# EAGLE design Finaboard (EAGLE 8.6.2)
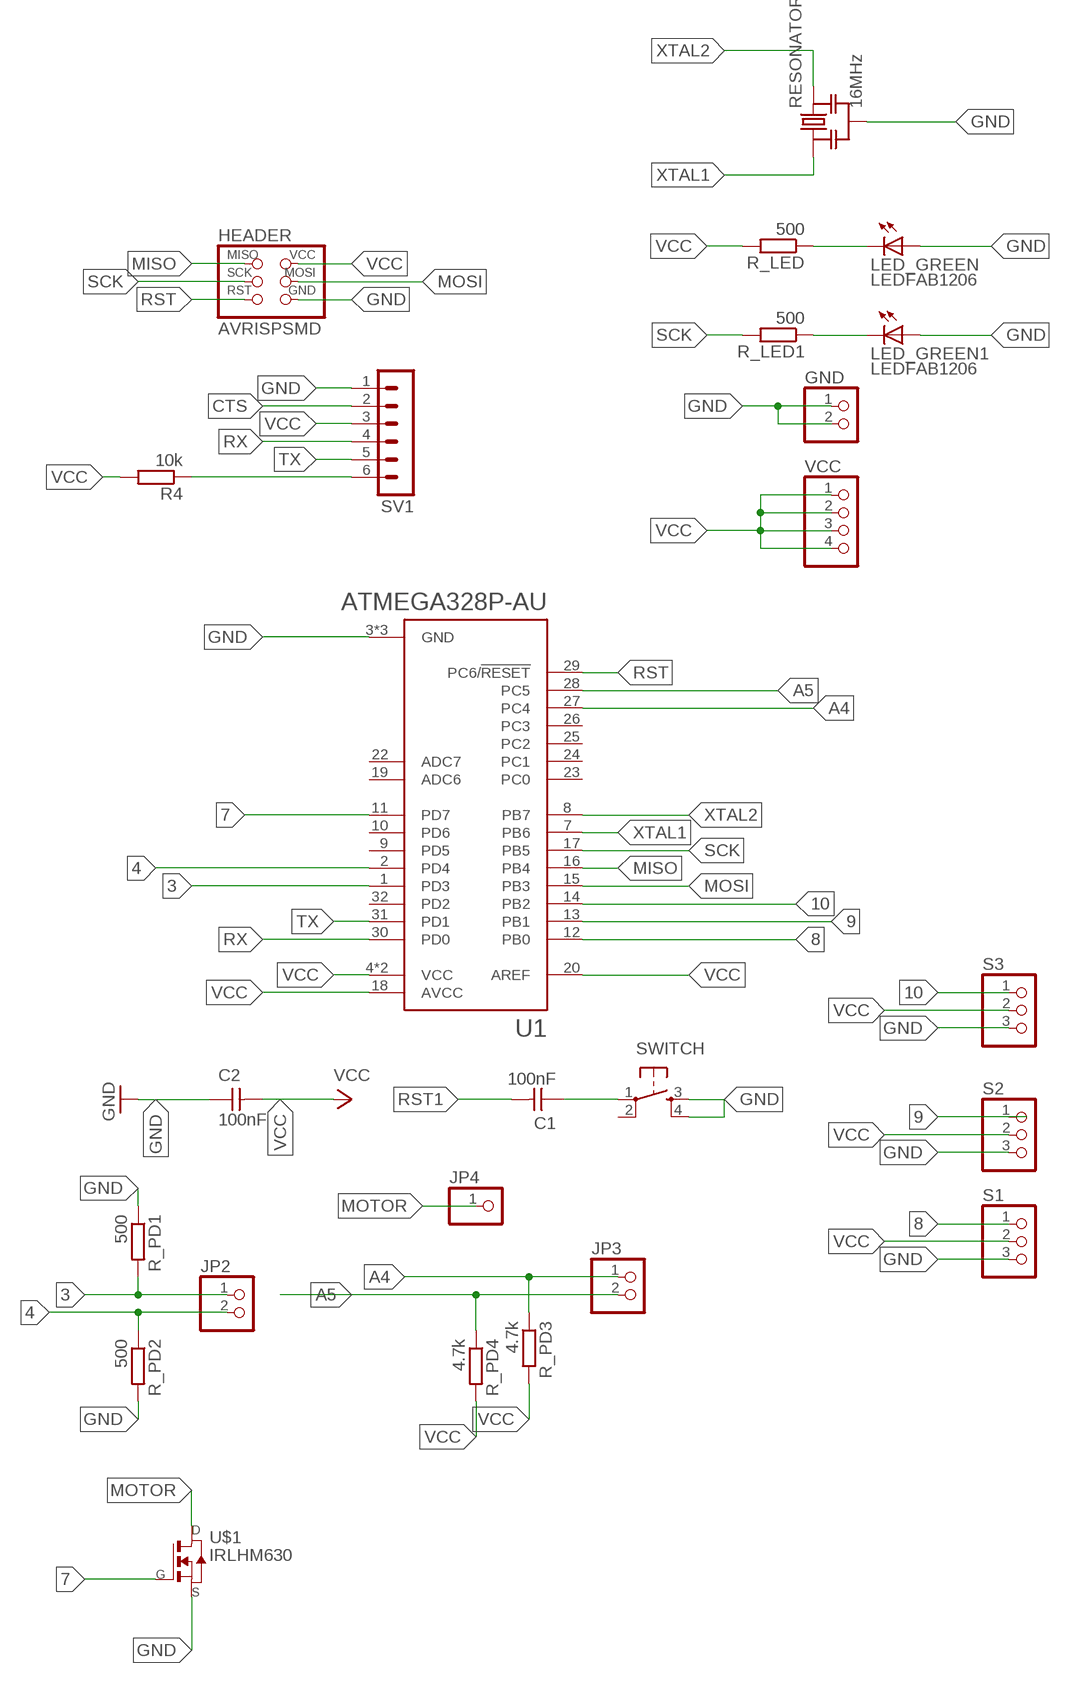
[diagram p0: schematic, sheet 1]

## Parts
C1  100nF  CAP-UNPOLARIZEDFAB  [C1206FAB]
C2  100nF  CAP-UNPOLARIZEDFAB  [C1206FAB]
GND  PINHD-1X2  [1X02]
HEADER  AVRISPSMD  [2X03SMD]
JP2  PINHD-1X2  [1X02]
JP3  PINHD-1X2  [1X02]
JP4  PINHD-1X1  [1X01]
LED_GREEN  LEDFAB1206  [LED1206FAB]
LED_GREEN1  LEDFAB1206  [LED1206FAB]
R4  10k  R-EU_R1206  [R1206]
R_LED  500  R-EU_R1206  [R1206]
R_LED1  500  R-EU_R1206  [R1206]
R_PD1  500  R-EU_R1206  [R1206]
R_PD2  500  R-EU_R1206  [R1206]
R_PD3  4.7k  R-EU_R1206  [R1206]
R_PD4  4.7k  R-EU_R1206  [R1206]
RESONATOR  16MHz  RESONATOR-MURATACSTCR_G  [RESONATOR_MURATA3]
S1  PINHD-1X3  [1X03]
S2  PINHD-1X3  [1X03]
S3  PINHD-1X3  [1X03]
SV1  MA06-1  [MA06-1]
SWITCH  6MM_SWITCH6MM_SWITCH  [6MM_SWITCH]
U1  ATMEGA328P-AU  [QFP80P900X900X120-32N]
U$1  IRLHM630  [IRF-PQFN3.3X3.3B]
VCC  PINHD-1X4  [1X04]

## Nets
3: JP2.1 R_PD1.2 U1.1(PD3)
4: JP2.2 R_PD2.1 U1.2(PD4)
7: U1.11(PD7) U$1.G
8: S1.1 U1.12(PB0)
9: S2.1 U1.13(PB1)
10: S3.1 U1.14(PB2)
A4: JP3.1 R_PD3.1 U1.27(PC4)
A5: JP3.2 R_PD4.1 U1.28(PC5)
CTS: SV1.2
GND: C2.1 GND.1 GND.2 HEADER.6(GND) LED_GREEN1.1(A) LED_GREEN.1(A) R_PD1.1 R_PD2.2 RESONATOR.2 S1.3 S2.3 S3.3 SV1.1 SWITCH.3(S) SWITCH.4(S1) U1.3(GND) U1.5(GND) U1.21(GND) U$1.S
MISO: HEADER.1(MISO) U1.16(PB4)
MOSI: HEADER.4(MOSI) U1.15(PB3)
MOTOR: JP4.1 U$1.D
N$1: LED_GREEN1.2(C) R_LED1.1
N$21: LED_GREEN.2(C) R_LED.1
RST: C1.1 HEADER.5(RST) SWITCH.1(P) U1.29(PC6/!RESET)
RST1: C1.2 R4.1 SV1.6
RX: SV1.4 U1.30(PD0)
SCK: HEADER.3(SCK) R_LED1.2 U1.17(PB5)
TX: SV1.5 U1.31(PD1)
VCC: C2.2 HEADER.2(VCC) R4.2 R_LED.2 R_PD3.2 R_PD4.2 S1.2 S2.2 S3.2 SV1.3 U1.4(VCC) U1.6(VCC) U1.18(AVCC) U1.20(AREF) VCC.1 VCC.2 VCC.3 VCC.4
XTAL1: RESONATOR.1 U1.7(PB6)
XTAL2: RESONATOR.3 U1.8(PB7)
Unconnected: SWITCH.2(P1) U1.9(PD5) U1.10(PD6) U1.19(ADC6) U1.22(ADC7) U1.23(PC0) U1.24(PC1) U1.25(PC2) U1.26(PC3) U1.32(PD2)

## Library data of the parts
C1 C2 = fab:CAP-UNPOLARIZED
GND JP2 JP3 = pinhead:PINHD-1X2: PIN HEADER
HEADER = fab:AVRISP
JP4 = pinhead:PINHD-1X1: PIN HEADER
LED_GREEN LED_GREEN1 = fab:LED: LED
R4 R_LED R_LED1 R_PD1-R_PD4 = resistor:R-EU_: RESISTOR, European symbol
RESONATOR = m-pad-2.1:RESONATOR-MURATA: Murata ceramic Resonator "ceralock" CSTCE series with built in load capacitance +- 0.5% tolerance 12.51MHz to 19.99MHz 16MHz murata part#: CSTCE16M0V53-R0 16MHz digikey part#: 490-1198-1-ND $1.33 each
S1-S3 = pinhead:PINHD-1X3: PIN HEADER
SV1 = con-lstb:MA06-1: PIN HEADER; OC_FARNELL: unknown; OC_NEWARK: unknown
SWITCH = fab:6MM_SWITCH: OMRON SWITCH
U1 = ATMEGA328P-AU:ATMEGA328P-AU: ATmega Series 20 MHz 32 KB Flash 2 KB SRAM 8-Bit Microcontroller - TQFP-32; AVAILABILITY: Good; DESCRIPTION: ATmega Series 20 MHz 32 KB Flash 2 KB SRAM 8-Bit Microcontroller - TQFP-32; MF: Atmel; MP: ATMEGA328P-AU; PACKAGE: TQFP-32 Atmel; PRICE: 2.38 USD
U$1 = fab:IRLHM630
VCC = pinhead:PINHD-1X4: PIN HEADER

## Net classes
0 default: clearance 0.205 mm

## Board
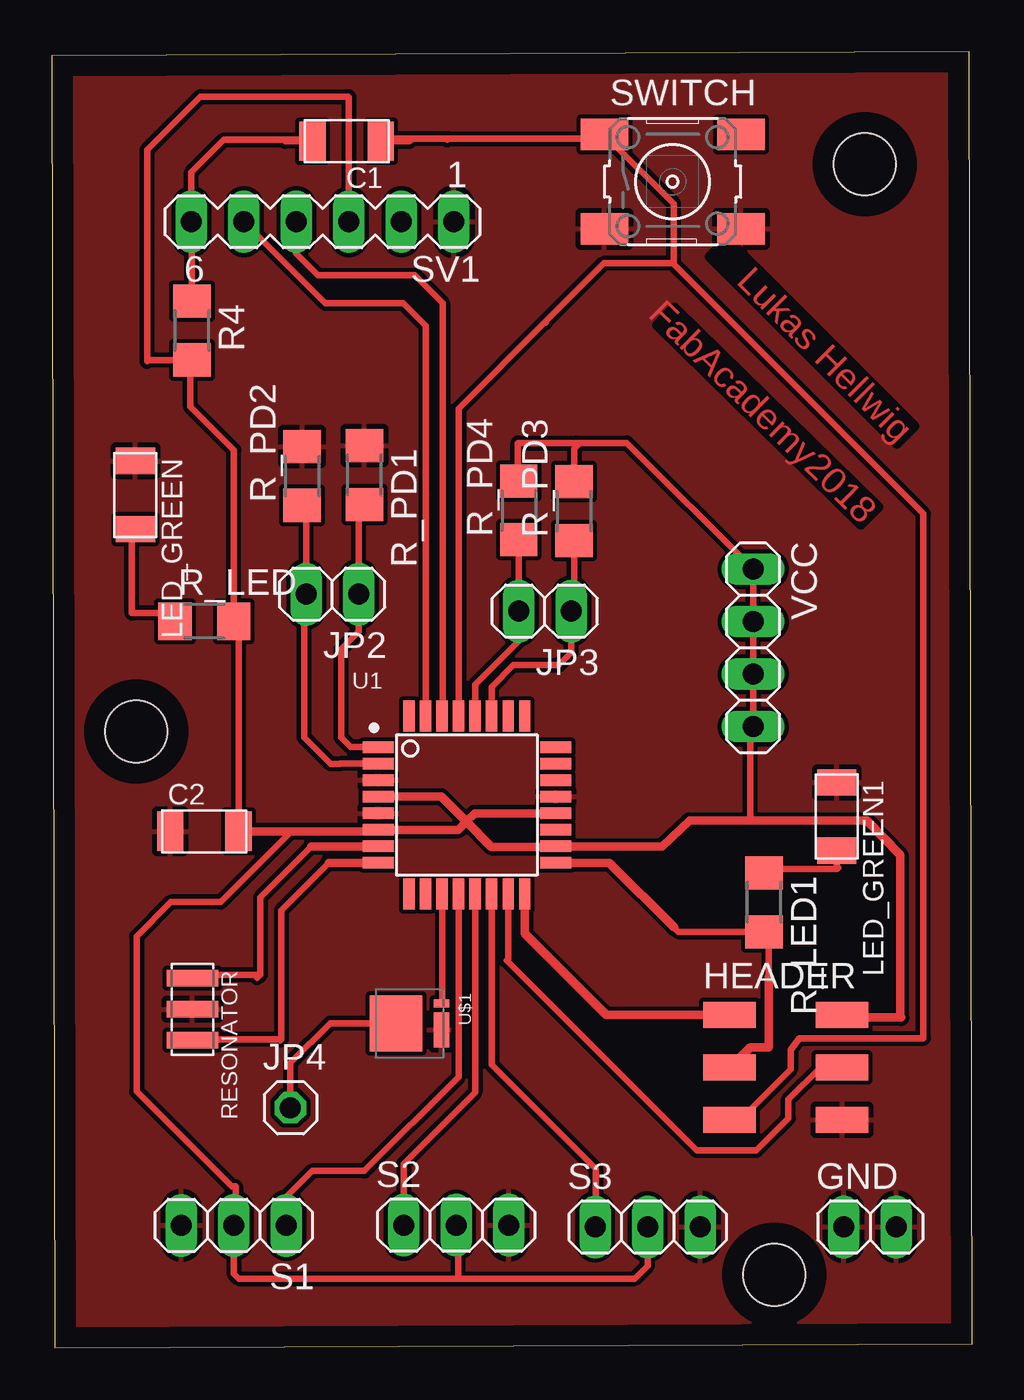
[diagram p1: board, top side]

Size 44.53 x 62.74 mm. Coordinates in mm from the lower left corner, seen from the top.
Outline: 0.14,0 44.53,0.2 44.39,62.74 0,62.54 0.14,0
Copper layers (1*16): Top 0.035mm / dielectric 1.5mm / Bottom 0.035mm
Design rules "default *": minimum track width 6mil, minimum drill 0.35mm, track to track 8mil, track to pad 8mil, pad to pad 8mil, via to via 8mil, smd to smd 8mil, copper to edge 40mil, drill to drill 8mil, minimum pad ring 10mil, minimum via ring 8mil, stop-mask expansion 4mil, vias tented up to drill 0mil, thermal gap 10mil
Holes 3 mm at 39.34,57.3 34.96,3.54 4.09,29.84

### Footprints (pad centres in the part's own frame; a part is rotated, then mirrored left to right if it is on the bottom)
C1206FAB = smd 1.27 x 1.905: 1 -1.651,0; 2 1.651,0
1X02 = drill 1.016 long: 1 -1.27,0; 2 1.27,0
2X03SMD = smd 2.54 x 1.27: 1 -2.54,2.54; 2 2.92,2.54; 3 -2.54,0; 4 2.92,0; 5 -2.54,-2.54; 6 2.92,-2.54
1X01 = drill 1.016 octagon: 1 0,0
LED1206FAB = smd 1.27 x 1.905: 1 -1.651,0; 2 1.651,0
R1206 = smd 1.6 x 1.803: 1 -1.422,0; 2 1.422,0
RESONATOR_MURATA3 = smd 0.8 x 2.5: 1 -1.5,0; 2 0,0; 3 1.5,0
1X03 = drill 1.016 long: 1 -2.54,0; 2 0,0; 3 2.54,0
MA06-1 = drill 1.016 long: 1 -6.35,0; 2 -3.81,0; 3 -1.27,0; 4 1.27,0; 5 3.81,0; 6 6.35,0
6MM_SWITCH = smd 2.286 x 1.524: 1 -3.302,2.286; 2 3.302,2.286; 3 -3.302,-2.286; 4 3.302,-2.286
QFP80P900X900X120-32N = smd 1.5 x 0.55: 1 -4.3,2.8; 2 -4.3,2; 3 -4.3,1.2; 4 -4.3,0.4; 5 -4.3,-0.4; 6 -4.3,-1.2; 7 -4.3,-2; 8 -4.3,-2.8; 17 4.3,-2.8; 18 4.3,-2; 19 4.3,-1.2; 20 4.3,-0.4; 21 4.3,0.4; 22 4.3,1.2; 23 4.3,2; 24 4.3,2.8 | smd 0.55 x 1.5: 9 -2.8,-4.3; 10 -2,-4.3; 11 -1.2,-4.3; 12 -0.4,-4.3; 13 0.4,-4.3; 14 1.2,-4.3; 15 2,-4.3; 16 2.8,-4.3; 25 2.8,4.3; 26 2,4.3; 27 1.2,4.3; 28 0.4,4.3; 29 -0.4,4.3; 30 -1.2,4.3; 31 -2,4.3; 32 -2.8,4.3
IRF-PQFN3.3X3.3B = smd 2.7 x 2.54: D 0,-1.27 | smd 0.39 x 0.77: G -0.975,0.925 | smd 1.69 x 0.77: S 0.325,0.925
1X04 = drill 1.016 long: 1 -3.81,0; 2 -1.27,0; 3 1.27,0; 4 3.81,0

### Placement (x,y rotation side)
C1  14.27,58.41 180 top
C2  7.39,25.01 0 top
GND  39.6,5.85 0 top
HEADER  35.33,13.58 0 top
JP2  13.58,36.48 180 top
JP3  23.87,35.65 180 top
JP4  11.55,11.63 0 top
LED_GREEN  4.05,41.28 270 top
LED_GREEN1  37.99,25.72 270 top
R4  6.79,49.25 270 top
R_LED  7.39,35.17 0 top
R_LED1  34.47,21.56 270 top
R_PD1  15.13,42.25 270 top
R_PD2  12.12,42.21 90 top
R_PD3  25.28,40.5 90 top
R_PD4  22.6,40.54 90 top
RESONATOR  6.81,16.39 270 top
S1  8.81,5.93 180 top
S2  19.57,5.94 0 top
S3  28.84,5.85 0 top
SV1  13.11,54.51 180 top
SWITCH  30.05,56.45 0 top
U1  20.09,26.28 0 top
U$1  17.94,15.71 270 top
VCC  33.94,33.88 270 top

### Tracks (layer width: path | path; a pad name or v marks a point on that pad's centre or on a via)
3
  Top 0.305: U1.1 14.48,29.08 14,29.55 14,33.83 14.85,34.68 JP2.1 14.85,40.55 R_PD1.2
4
  Top 0.305: U1.2 13.96,28.28 13.95,28.27 13.49,28.27 12.21,29.55 12.21,36.38 JP2.2 12.31,40.59 R_PD2.1
7
  Top 0.305: U1.11 18.89,16.71 U$1.G
8
  Top 0.305: U1.12 19.69,13.13 15.13,8.56 12.61,8.56 11.35,7.31 S1.1
9
  Top 0.305: U1.13 20.49,12.38 17.03,8.92 S2.1
10
  Top 0.305: U1.14 21.29,13.71 26.33,8.67 26.33,5.88 S3.1
A4
  Top 0.305: U1.27 21.29,32 22.35,33.05 24.54,33.05 25.14,33.65 JP3.1 25.28,35.79 R_PD3.1
A5
  Top 0.305: U1.28 20.49,32.11 22.6,34.21 JP3.2 R_PD4.1
GND
  pour Top: -45.95,83.43 -45.95,-52.46 -44.68,-53.73 70.89,-53.73 77.24,-47.38 77.24,84.7 67.08,94.86 -34.52,94.86
MISO
  Top 0.406: U1.16 22.89,20.07 26.84,16.12 HEADER.1
MOSI
  Top 0.305: HEADER.4 37.21,13.58 35.65,12.02 35.65,11.12 34.09,9.55 31.22,9.55 22.03,18.75 22.09,18.82 U1.15
  Top 0.406: HEADER.4 38.26,13.57
MOTOR
  Top 0.305: U$1.D 13.47,15.71 11.55,13.79 JP4.1
N$1
  Top 0.305: R_LED1.1 34.67,23.18 38.02,23.18 38.07,23.23 37.99,23.32 LED_GREEN1.2
N$21
  Top 0.305: R_LED.1 5.57,35.57 3.88,35.57 3.88,39.46 LED_GREEN.2
  Top 0.406: R_LED.1 6.12,35.32
RST
  Top 0.152: 26.4,58.74 SWITCH.1 27.04,58.44
  Top 0.305: 19.13,58.48 19.19,58.53 | 19.19,58.53 26.2,58.53 26.4,58.74 | 30.1,52.5 30.1,52.66 30.1,55.39 27.04,58.44 | 30.1,52.5 26.72,52.5 23.87,49.65 | 23.87,49.65 23.9,49.62 | HEADER.5 33.31,11.04 35.76,13.48 35.76,14.42 36.19,14.98 42.18,14.98 42.18,40.38 30.1,52.47 30.1,52.5 | 19.19,58.53 17.44,58.53 | 17.44,58.53 16.05,58.53 | C1.1 17.31,58.41 17.44,58.53 | 23.87,49.65 19.69,45.48 U1.29
RST1
  Top 0.305: 6.76,54.64 SV1.6 6.79,54.48 R4.1 | 6.76,54.64 6.76,56.91 8.33,58.48 11.22,58.48 | 11.22,58.48 12.55,58.48 | 6.79,54.61 6.76,54.64 | C1.2 11.29,58.41 11.22,58.48
RX
  Top 0.305: SV1.4 11.84,52.96 12.88,51.92 17.57,51.92 17.64,51.85 18.92,50.56 18.92,30.61 U1.30
SCK
  Top 0.305: 30.12,20.35 30.33,20.14 R_LED1.2 34.69,19.93 34.69,17.97
  Top 0.406: U1.17 26.99,23.48 30.12,20.35 | HEADER.3 32.8,13.57 33.79,14.56 34.69,14.56 34.69,17.97
TX
  Top 0.305: SV1.5 13.25,50.56 17.02,50.56 18.09,49.49 U1.31
VCC
  Top 0.305: C2.2 9.04,34.94 R_LED.2 8.81,43.46 6.72,45.56 6.72,47.75 R4.2 4.69,47.82 4.62,47.76 4.62,58 7.2,60.57 14.35,60.57 14.38,60.54 SV1.3 | R_PD4.2 22.56,42.01 22.56,43.8 25.39,43.8 | 25.39,43.8 25.47,43.72 25.28,43.52 R_PD3.2 | 25.39,43.8 27.83,43.8 VCC.1 VCC.2 VCC.3 VCC.4 33.79,29.92 33.79,25.53 | 19.67,3.35 9.06,3.35 8.81,3.59 S1.2 8.9,6.01 8.9,7.81 8.71,7.81 4.11,12.41 4.11,19.93 5.77,21.58 8.17,21.58 11.6,25.01 | 19.67,3.35 28.2,3.35 28.84,3.98 S3.2 | 19.67,3.35 19.67,5.84 S2.2
  Top 0.406: U1.4 18.86,26.68 20.07,25.47 | 20.07,25.47 21.28,24.26 24.37,24.26 U1.18 29.55,24.28 30.87,25.53 33.79,25.53 39.44,25.53 41.05,23.85 41.05,16.04 41.1,15.99 38.38,15.99 HEADER.2 | 20.07,25.47 19.67,25.08 U1.6 15.72,25.01 11.6,25.01 C2.2 | U1.20 20.47,25.88 20.07,25.47
XTAL1
  Top 0.305: 12.57,24.28 10.09,21.8 10.09,18.06 | 10.09,18.06 9.95,17.91 | 10.09,18.06 6.98,18.06 RESONATOR.1
  Top 0.406: U1.7 12.57,24.28
XTAL2
  Top 0.305: 13.41,23.48 11.11,21.18 11.11,14.94 | 11.11,14.94 11.06,14.89 | 11.11,14.94 6.86,14.94 RESONATOR.3
  Top 0.406: U1.8 13.41,23.48

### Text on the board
Top: Lukas Hellwig | FabAcademy2018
